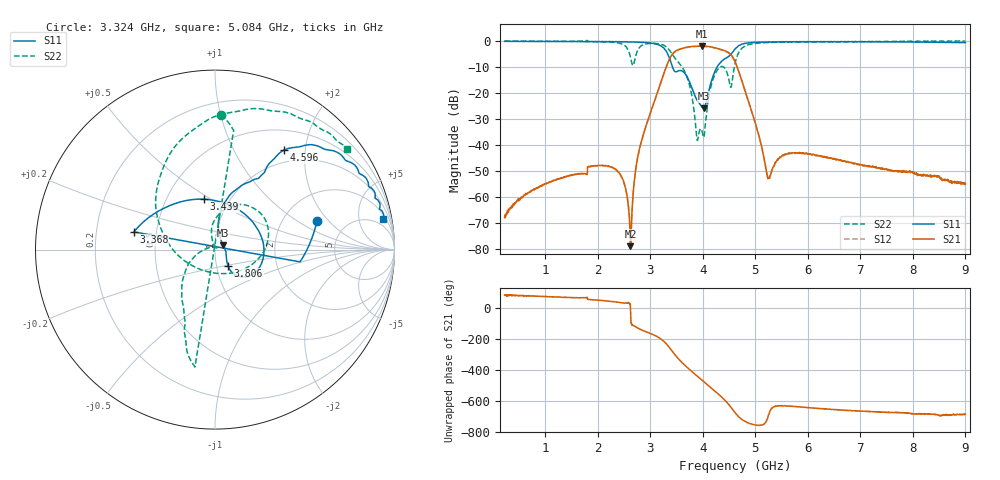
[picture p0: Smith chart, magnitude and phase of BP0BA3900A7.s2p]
!Agilent Technologies,E8358A,US41080443,A.07.50.56
!Agilent E8358A: A.07.50.56
!Date: Friday, December 15, 2017 21:17:43
!Correction: S11(Full 2 Port(1,2))
!S21(Full 2 Port(1,2))
!S12(Full 2 Port(1,2))
!S22(Full 2 Port(1,2))
!S2P File: Measurements: S11, S21, S12, S22:
# Hz S  dB  R 50
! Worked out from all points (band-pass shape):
!   1601 points, 225 MHz to 9 GHz, reference 50 ohm
!   highest |S21| = -1.91 dB at 3.987 GHz (marker M1); lowest = -78.8 dB at 2.622 GHz (marker M2)
!   |S21| within 3 dB of the highest: 3.424 GHz to 4.521 GHz (1.098 GHz wide, 27.6 % of centre)
!   lowest |S11| = -25.7 dB at 4.015 GHz (marker M3), VSWR 1.11, Z = 54.7 + j2.62 ohm
!   |S11| at or under -10 dB: 3.422 GHz to 4.27 GHz (847.7 MHz wide, 22 % of centre)
!   |S22| runs from -38.2 to 0.3 dB; largest |S21 - S12| = 0.011
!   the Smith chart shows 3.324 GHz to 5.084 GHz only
!   S11 on the Smith chart (normalised r, x): 3.324 GHz: 3.08, +1.49; 3.368 GHz: 0.37, +0.09; 3.439 GHz: 0.76, +0.47; 3.806 GHz: 1.14, -0.21; 4.596 GHz: 0.79, +1.61; 5.084 GHz: 3, +10
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2.25e8  -0.06 176.8  -67.67 82.1  -67.91 82.9  -0.00 175.9
1.689328e9  -0.14 149.0  -50.93 64.6  -50.93 63.9  0.05 162.6
2.363906e9  -0.23 140.2  -49.75 35.8  -49.72 36.3  -0.62 107.9
2.621672e9  -0.29 129.7  -78.79 0.1  -75.95 -1.7  -6.15 21.1
2.703938e9  -0.41 125.5  -52.05 -119.7  -52.11 -119.1  -7.10 -115.0
2.813625e9  -0.43 118.3  -39.70 -140.7  -39.76 -140.3  -2.00 173.5
3.153656e9  -1.42 76.1  -18.67 169.5  -18.73 169.4  -1.01 115.4
3.323672e9  -4.60 15.5  -8.78 120.5  -8.85 120.9  -2.51 87.6
3.367547e9  -6.69 167.7  -6.75 102.4  -6.89 102.6  -3.56 -99.7
3.438844e9  -10.83 102.3  -4.56 70.2  -4.67 70.6  -5.65 -108.4
3.806297e9  -18.74 -51.0  -2.02 -55.7  -2.14 -55.6  -22.98 -175.4
3.987281e9  -25.42 9.3  -1.91 -106.9  -2.03 -106.9  -34.94 24.2
4.014703e9  -25.74 27.5  -1.94 -114.6  -2.03 -114.4  -36.95 57.3
4.245047e9  -11.00 77.2  -2.61 178.9  -2.70 179.0  -12.13 72.1
4.596047e9  -3.43 55.3  -7.09 51.8  -7.24 51.7  -10.34 162.6
4.6125e9  -3.01 53.3  -7.79 44.3  -7.94 44.7  -8.67 150.6
4.782516e9  -0.96 33.0  -17.72 -8.1  -17.87 -8.3  -2.18 81.2
5.084156e9  -0.44 10.5  -37.62 -37.6  -37.64 -37.7  -0.70 37.2
5.254172e9  -0.27 3.3  -52.65 29.8  -52.45 31.8  -0.50 24.3
6.076828e9  -0.27 -20.6  -43.67 74.7  -43.63 74.3  -0.32 -14.9
7.541156e9  -0.24 -49.4  -49.40 46.7  -49.40 47.2  -0.12 -48.1
9e9  -0.54 -95.6  -54.76 35.3  -54.79 33.2  0.06 -42.9
